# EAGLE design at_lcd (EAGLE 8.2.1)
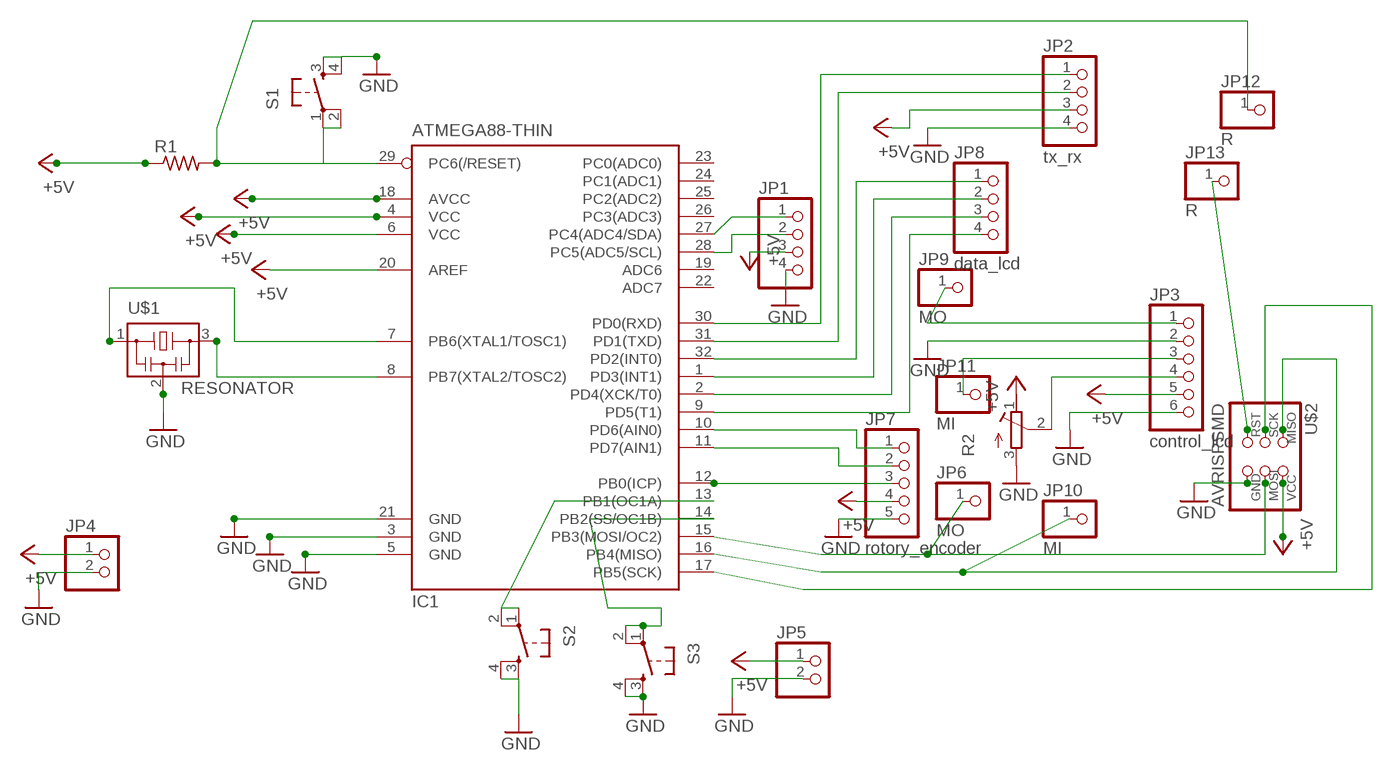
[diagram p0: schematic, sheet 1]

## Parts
IC1  ATMEGA88-THIN  [TQFP32-08THIN]
JP1  PINHD-1X4  [1X04]
JP2  tx_rx  PINHD-1X4  [1X04]
JP3  control_lcd  PINHD-1X6  [1X06]
JP4  PINHD-1X2  [1X02]
JP5  PINHD-1X2  [1X02]
JP6  MO  PINHD-1X1  [1X01]
JP7  rotory_encoder  PINHD-1X5  [1X05]
JP8  data_lcd  PINHD-1X4  [1X04]
JP9  MO  PINHD-1X1  [1X01]
JP10  MI  PINHD-1X1  [1X01]
JP11  MI  PINHD-1X1  [1X01]
JP12  R  PINHD-1X1  [1X01]
JP13  R  PINHD-1X1  [1X01]
R1  RES-US1206FAB  [R1206FAB]
R2  R-TRIMMT93XB  [RTRIMT93XB]
S1  6MM_SWITCH6MM_SWITCH  [6MM_SWITCH]
S2  6MM_SWITCH6MM_SWITCH  [6MM_SWITCH]
S3  6MM_SWITCH6MM_SWITCH  [6MM_SWITCH]
U$1  RESONATOR  [EFOBM]
U$2  AVRISPSMD  [2X03SMD]

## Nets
+5V: IC1.4(VCC) IC1.6(VCC) IC1.18(AVCC) IC1.20(AREF) JP1.3 JP2.3 JP3.5 JP4.1 JP5.1 JP7.4 R1.1 R2.1(E) U$2.2(VCC)
GND: IC1.3(GND) IC1.5(GND) IC1.21(GND) JP1.4 JP2.4 JP3.2 JP3.6 JP4.2 JP5.2 JP7.5 R2.3(A) S1.3(S) S1.4(S1) S2.3(S) S2.4(S1) S3.3(S) S3.4(S1) U$1.2 U$2.6(GND)
N$1: IC1.7(PB6(XTAL1/TOSC1)) U$1.1
N$2: IC1.8(PB7(XTAL2/TOSC2)) U$1.3
N$3: IC1.13(PB1(OC1A)) S2.1(P) S2.2(P1)
N$4: IC1.17(PB5(SCK)) U$2.3(SCK)
N$5: IC1.16(PB4(MISO)) JP10.1 U$2.1(MISO)
N$6: IC1.15(PB3(MOSI/OC2)) JP6.1 U$2.4(MOSI)
N$7: IC1.32(PD2(INT0)) JP8.1
N$8: IC1.1(PD3(INT1)) JP8.2
N$9: IC1.2(PD4(XCK/T0)) JP8.3
N$10: IC1.9(PD5(T1)) JP8.4
N$11: JP3.4 R2.2(S)
N$12: IC1.14(PB2(SS/OC1B)) S3.1(P) S3.2(P1)
N$13: IC1.10(PD6(AIN0)) JP7.1
N$14: IC1.11(PD7(AIN1)) JP7.2
N$15: IC1.12(PB0(ICP)) JP7.3
N$16: IC1.30(PD0(RXD)) JP2.1
N$17: IC1.31(PD1(TXD)) JP2.2
N$18: IC1.28(PC5(ADC5/SCL)) JP1.2
N$19: IC1.27(PC4(ADC4/SDA)) JP1.1
N$20: IC1.29(PC6(/RESET)) JP12.1 R1.2 S1.1(P) S1.2(P1)
N$21: JP13.1 U$2.5(RST)
N$22: JP3.3 JP11.1
N$23: JP3.1 JP9.1
Unconnected: IC1.19(ADC6) IC1.22(ADC7) IC1.23(PC0(ADC0)) IC1.24(PC1(ADC1)) IC1.25(PC2(ADC2)) IC1.26(PC3(ADC3))

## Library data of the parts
IC1 = fab:ATMEGA88-THIN
JP1 JP2 JP8 = pinhead:PINHD-1X4: PIN HEADER
JP3 = pinhead:PINHD-1X6: PIN HEADER
JP4 JP5 = pinhead:PINHD-1X2: PIN HEADER
JP6 JP9-JP13 = pinhead:PINHD-1X1: PIN HEADER
JP7 = pinhead:PINHD-1X5: PIN HEADER
R1 = fab:RES-US: Resistor (US Symbol)
R2 = resistor:R-TRIMM: Trimm resistor
S1-S3 = fab:6MM_SWITCH: OMRON SWITCH
U$1 = fab:RESONATOR
U$2 = fab:AVRISP

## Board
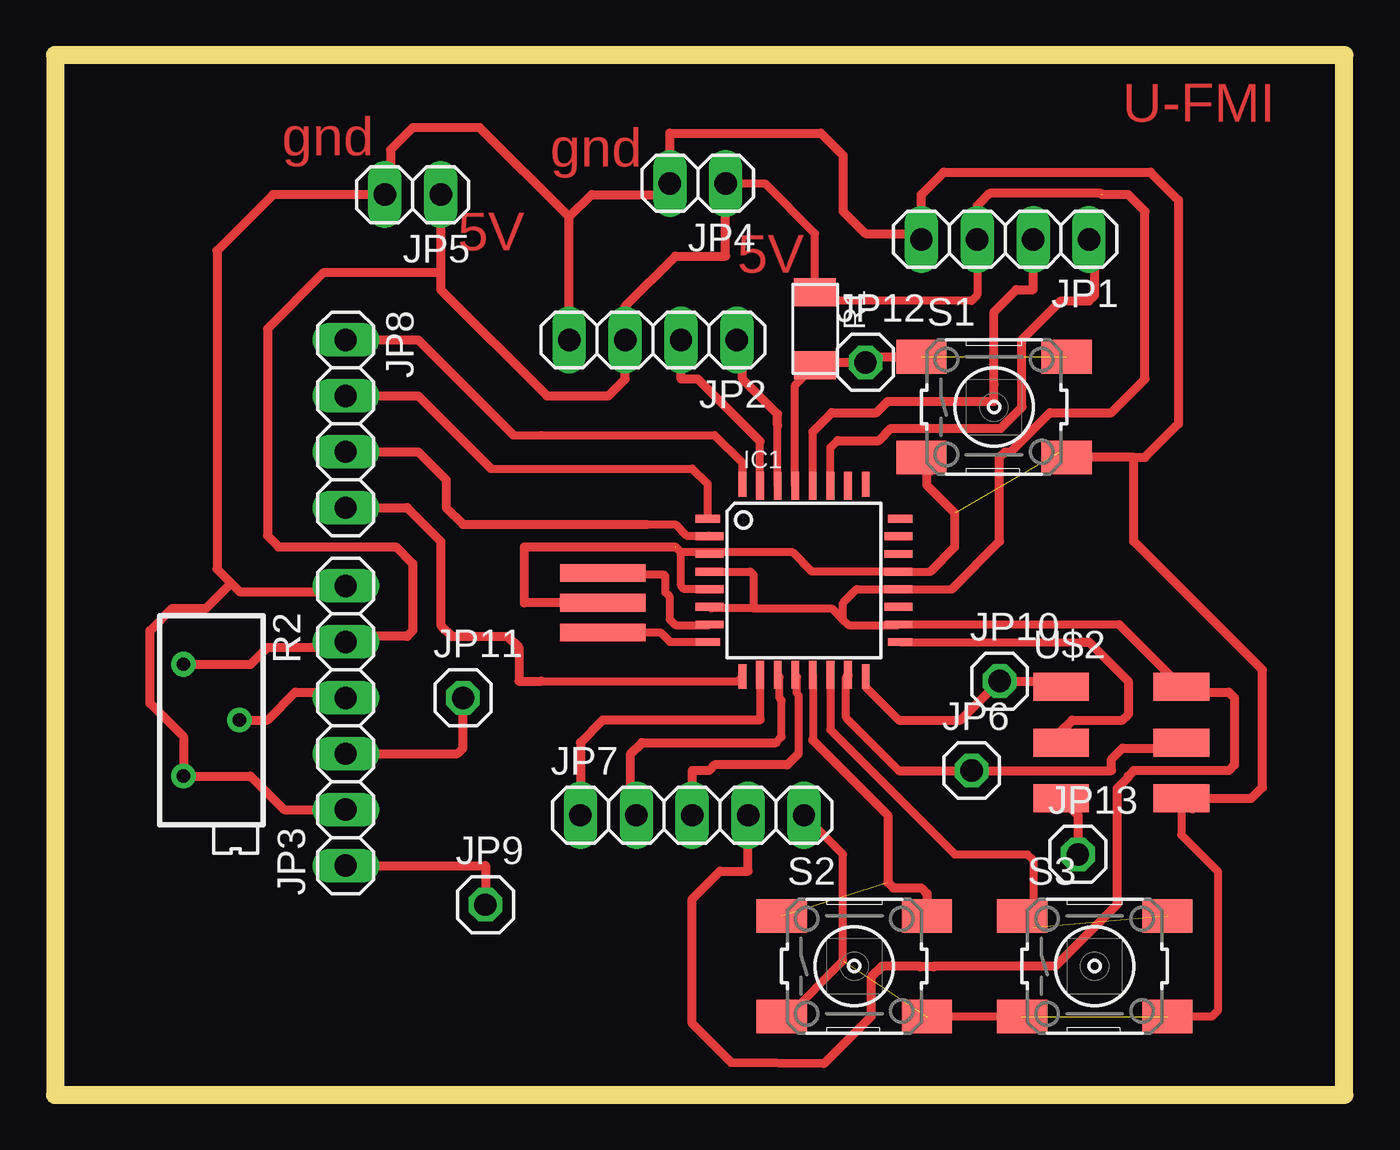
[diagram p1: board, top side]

Size 58.6 x 47.23 mm. Coordinates in mm from the lower left corner, seen from the top.
Outline: 0,0 58.6,0 58.6,47.23 0,47.23 0,0
Copper layers (1*16): Top 0.035mm / dielectric 1.5mm / Bottom 0.035mm
Design rules "default *": minimum track width 14mil, minimum drill 32mil, track to track 14mil, track to pad 14mil, pad to pad 14mil, via to via 14mil, smd to smd 14mil, copper to edge 40mil, drill to drill 8mil, minimum pad ring 10mil, minimum via ring 8mil, stop-mask expansion 4mil, vias tented up to drill 0mil, thermal gap 10mil

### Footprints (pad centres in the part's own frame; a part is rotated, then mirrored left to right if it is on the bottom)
TQFP32-08THIN = smd 1.118 x 0.356: 1 -4.369,2.8; 8 -4.369,-2.8; 17 4.369,-2.8; 24 4.369,2.8 | smd 1.27 x 0.356: 2 -4.293,2; 3 -4.293,1.2; 4 -4.293,0.4; 5 -4.293,-0.4; 6 -4.293,-1.2; 7 -4.293,-2; 18 4.293,-2; 19 4.293,-1.2; 20 4.293,-0.4; 21 4.293,0.4; 22 4.293,1.2; 23 4.293,2 | smd 0.356 x 1.118: 9 -2.8,-4.369; 16 2.8,-4.369; 25 2.8,4.369; 32 -2.8,4.369 | smd 0.356 x 1.27: 10 -2,-4.293; 14 1.2,-4.293; 15 2,-4.293; 26 2,4.293; 27 1.2,4.293; 31 -2,4.293 | smd 0.35 x 1.27: 11 -1.2,-4.293; 12 -0.4,-4.293; 13 0.4,-4.293; 28 0.4,4.293; 29 -0.4,4.293; 30 -1.2,4.293
1X04 = drill 1.016 long: 1 -3.81,0; 2 -1.27,0; 3 1.27,0; 4 3.81,0
1X06 = drill 1.016 long: 1 -6.35,0; 2 -3.81,0; 3 -1.27,0; 4 1.27,0; 5 3.81,0; 6 6.35,0
1X02 = drill 1.016 long: 1 -1.27,0; 2 1.27,0
1X01 = drill 1.016 octagon: 1 0,0
1X05 = drill 1.016 long: 1 -5.08,0; 2 -2.54,0; 3 0,0; 4 2.54,0; 5 5.08,0
R1206FAB = smd 1.27 x 1.905: 1 -1.651,0; 2 1.651,0
RTRIMT93XB = drill 0.61: 1 1.27,-2.54; 2 -1.27,0; 3 1.27,2.54
6MM_SWITCH = smd 2.286 x 1.524: 1 -3.302,2.286; 2 3.302,2.286; 3 -3.302,-2.286; 4 3.302,-2.286
EFOBM = smd 0.8 x 3.9: 1 -1.35,0; 2 0,0; 3 1.35,0
2X03SMD = smd 2.54 x 1.27: 1 -2.54,2.54; 2 2.92,2.54; 3 -2.54,0; 4 2.92,0; 5 -2.54,-2.54; 6 2.92,-2.54

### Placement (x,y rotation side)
IC1  34.04,23.37 0 top
JP1  43.18,38.86 180 top
JP2  27.18,34.29 180 top
JP3  13.21,16.76 90 top
JP4  29.21,41.4 180 top
JP5  16.26,40.89 180 top
JP6  41.66,14.73 0 top
JP7  28.96,12.7 0 top
JP8  13.21,30.48 270 top
JP9  19.56,8.64 0 top
JP10  42.93,18.8 0 top
JP11  18.54,18.03 0 top
JP12  36.83,33.27 0 top
JP13  46.48,10.92 0 top
R1  34.54,34.8 270 top
R2  7.11,17.02 180 top
S1  42.67,31.24 0 top
S2  36.32,5.84 0 top
S3  47.24,5.84 0 top
U$1  24.89,22.35 270 top
U$2  48.26,16 0 top

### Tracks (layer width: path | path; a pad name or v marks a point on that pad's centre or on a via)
+5V  (1 unrouted)
  Top 0.356: IC1.4 31.6,23.77 31.75,23.62 31.75,22.1 | 31.75,22.1 29.81,22.1 IC1.6 | 35.81,21.59 35.81,22.35 36.43,22.97 IC1.20 40.75,22.97 | 35.81,21.59 36.07,21.34 38.3,21.34 IC1.18 48.35,21.37 | 31.75,22.1 35.31,22.1 35.81,21.59 | 47.55,40.89 47.53,40.92 | 42.16,39.12 JP1.3 41.91,36.32 41.66,36.07 34.92,36.07 R1.1 34.54,39.12 32.26,41.4 JP4.1 | JP5.1 17.27,40.64
  Top 0.406: JP5.1 17.53,37.34 | 17.53,37.34 12.19,37.34 9.65,34.8 9.65,25.4 10.16,24.89 15.49,24.89 16.26,24.13 16.26,21.08 16,20.83 13.46,20.83 JP3.5 12.95,20.32 9.65,20.32 8.89,19.56 R2.1 | 48.35,21.37 U$2.2 51.43,18.29 53.34,18.29 53.59,18.03 53.59,14.99 53.34,14.73 49.02,14.73 48.77,14.48 48.77,14.42 48.26,13.91 48.26,8.64 45.47,5.84 39.95,5.84 39.93,5.82 39.32,5.82 39.29,5.84 37.59,5.84 37.08,5.33 37.08,3.56 34.94,1.41 30.74,1.46 28.96,3.25 28.96,8.89 30.23,10.16 31.5,10.16 JP7.4 | 17.53,37.34 17.53,36.58 22.35,31.75 25.15,31.75 25.91,32.51 JP2.3 25.91,35.81 28.19,38.1 30.48,38.1 JP4.1 | 40.75,22.97 42.93,25.15 42.93,28.96 43.18,29.21 43.43,29.21 45.21,30.99 48.01,30.99 49.53,32.51 49.53,40.13 48.77,40.89 47.59,40.89 47.54,40.95 42.47,40.95 41.91,40.39 JP1.3
GND  (4 unrouted)
  Top 0.356: 22.86,22.35 U$1.2 | 28.45,24.64 28.19,24.89 | 29.67,24.64 28.45,24.64 | 29.67,24.64 IC1.3 | IC1.5 28.59,22.97 28.45,23.11 28.45,24.64 | 29.67,24.64 33.53,24.64 34.4,23.77 IC1.21 39.77,23.77 | 45.72,29.21 S1.4 | 39.88,28.45 S1.3 | 39.62,39.12 JP1.4 39.37,39.12 | 23.62,34.54 JP2.4 | 51.69,12.95 U$2.6 51.18,11.81 52.83,10.16 52.83,3.81 52.58,3.56 S3.4 | S3.3 S2.4 | S2.3 33.27,3.56 35.81,6.1 35.81,10.92 JP7.5
  Top 0.406: 8,23.24 7.37,23.88 7.37,38.35 9.91,40.89 JP5.2 15.24,41.15 15.24,42.93 16.26,43.94 19.3,43.94 23.37,39.88 | 8,23.24 8.38,22.86 12.95,22.86 JP3.6 | 8,23.24 6.86,22.1 5.33,22.1 4.32,21.08 4.32,17.78 5.84,16.26 R2.3 8.89,14.48 10.41,12.95 JP3.2 | U$2.6 54.36,13.46 54.86,13.97 54.86,19.3 49.02,25.15 49.02,28.96 | 49.02,28.96 S1.4 | 49.02,28.96 49.53,28.96 51.05,30.48 51.05,40.64 49.78,41.91 40.39,41.91 39.37,40.89 JP1.4 39.12,39.12 36.83,39.12 35.81,40.13 35.81,42.67 34.8,43.69 27.94,43.69 JP4.2 27.43,40.89 24.38,40.89 23.37,39.88 | JP2.4 23.37,39.88 | 39.77,23.77 40.89,24.89 40.89,26.42 39.62,27.69 39.62,28.19 39.88,28.45 | U$1.2 21.34,22.35 21.34,24.89 28.17,24.89
N$1
  Top 0.356: IC1.7 29.71,21.34 28.19,21.34 27.94,21.59 27.94,22.62 27.74,22.82 27.74,23.57 27.69,23.62 24.97,23.62 U$1.1
N$2
  Top 0.356: U$1.3 27.51,21 27.94,20.57 IC1.8
N$3  (1 unrouted)
  Top 0.356: IC1.13 34.44,16.11
  Top 0.406: 34.44,16.11 37.85,12.7 37.85,9.65 38.1,9.4 39.37,9.4 39.62,9.14 S2.2
N$4
  Top 0.356: IC1.17 46.74,20.57 | 46.1,15.87 46.23,15.75
  Top 0.406: 46.1,15.87 45.97,16 U$2.3 45.72,16.51 46.23,17.02 48.51,17.02 48.77,17.27 48.77,18.8 47,20.57 46.74,20.57
N$5
  Top 0.356: IC1.16 36.84,18.54 38.35,17.02 | U$2.1 45.47,18.8
  Top 0.406: 38.35,17.02 41.15,17.02 JP10.1 45.47,18.8 U$2.1
N$6
  Top 0.356: 38.35,14.73 35.95,17.14 35.95,18.99 IC1.15
  Top 0.406: 38.35,14.73 JP6.1 48.01,14.73 48.01,15.24 48.51,15.75 50.93,15.75 U$2.4 | IC1.15 35.97,18.77 35.97,18.64
N$7
  Top 0.356: 31.24,28.7 IC1.32 31.24,28.71 29.97,29.97 22.1,29.97 20.83,29.97
  Top 0.406: JP8.1 16.51,34.29 20.83,29.97
N$8
  Top 0.356: IC1.1 29.67,27.74 28.96,28.45 19.81,28.45 | 13.46,32 JP8.2
  Top 0.406: JP8.2 16.51,31.75 19.81,28.45
N$9
  Top 0.356: 26.92,25.91 28.19,25.91 28.7,25.4 29.71,25.4 IC1.2
  Top 0.406: JP8.3 15.49,29.21 | 15.49,29.21 15.75,29.21 | 15.49,29.21 16.51,29.21 17.78,27.94 17.78,26.67 18.54,25.91 26.92,25.91
N$10
  Top 0.356: 22.1,18.8 31.03,18.8 IC1.9
  Top 0.406: 22.1,18.8 21.08,18.8 21.08,20.32 20.57,20.83 18.03,20.83 17.53,21.34 17.53,25.15 16,26.67 JP8.4
N$11
  Top 0.406: R2.2 9.65,17.02 10.92,18.29 12.95,18.29 JP3.4
N$12  (1 unrouted)
  Top 0.356: IC1.14 35.24,16.58 40.89,10.92 44.2,10.92 44.45,10.67 44.45,7.62 S3.1
N$13
  Top 0.356: IC1.10 32.04,17.05 32,17.02 | JP7.1 24.13,12.95
  Top 0.406: 32.04,17.05 32,17.02 24.89,17.02 23.88,16 JP7.1
N$14
  Top 0.356: 32.77,16 33.02,16.26 33.02,17.92 32.92,18.02 32.92,18.99 IC1.11
  Top 0.406: JP7.2 26.16,12.95 26.16,15.49 26.67,16 32.77,16
N$15
  Top 0.356: 33.78,15.49 33.78,18.16 33.73,18.22 33.73,18.98 IC1.12
  Top 0.406: 33.78,15.49 33.27,14.99 29.97,14.99 29.72,14.73 28.96,14.73 JP7.3
N$16
  Top 0.356: IC1.30 32.84,30.41
  Top 0.406: 32.84,30.41 32.84,30.92 31.24,32.51 31.24,34.04 JP2.1
N$17
  Top 0.356: IC1.31 32.04,29.69
  Top 0.406: 32.04,29.69 29.21,32.51 28.45,32.51 JP2.2
N$18
  Top 0.356: IC1.28 34.44,30.12
  Top 0.406: 34.44,30.12 35.31,30.99 37.34,30.99 37.85,31.5 42.67,31.5 42.67,32.26 42.67,35.56 43.69,36.58 44.45,36.58 JP1.2
N$19
  Top 0.356: IC1.27 35.24,29.39 35.56,29.72
  Top 0.406: 35.56,29.72 37.44,29.72 38,30.28 42.98,30.28 43.94,31.24 43.94,34.29 45.72,36.07 46.99,36.07 47.24,36.32 47.24,38.61 JP1.1
N$20  (1 unrouted)
  Top 0.356: IC1.29 33.64,32.24 R1.2 34.67,33.27 | 38.99,33.15 S1.1 39.12,33.27
  Top 0.406: R1.2 34.67,33.27 JP12.1 37.08,33.53 S1.1
N$21
  Top 0.406: U$2.5 46.48,12.7 JP13.1
N$22
  Top 0.406: JP3.3 18.29,15.49 18.54,15.75 JP11.1
N$23
  Top 0.406: JP3.1 19.56,10.41 JP9.1

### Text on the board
Top: gnd | gnd | U-FMI | 5V | 5V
